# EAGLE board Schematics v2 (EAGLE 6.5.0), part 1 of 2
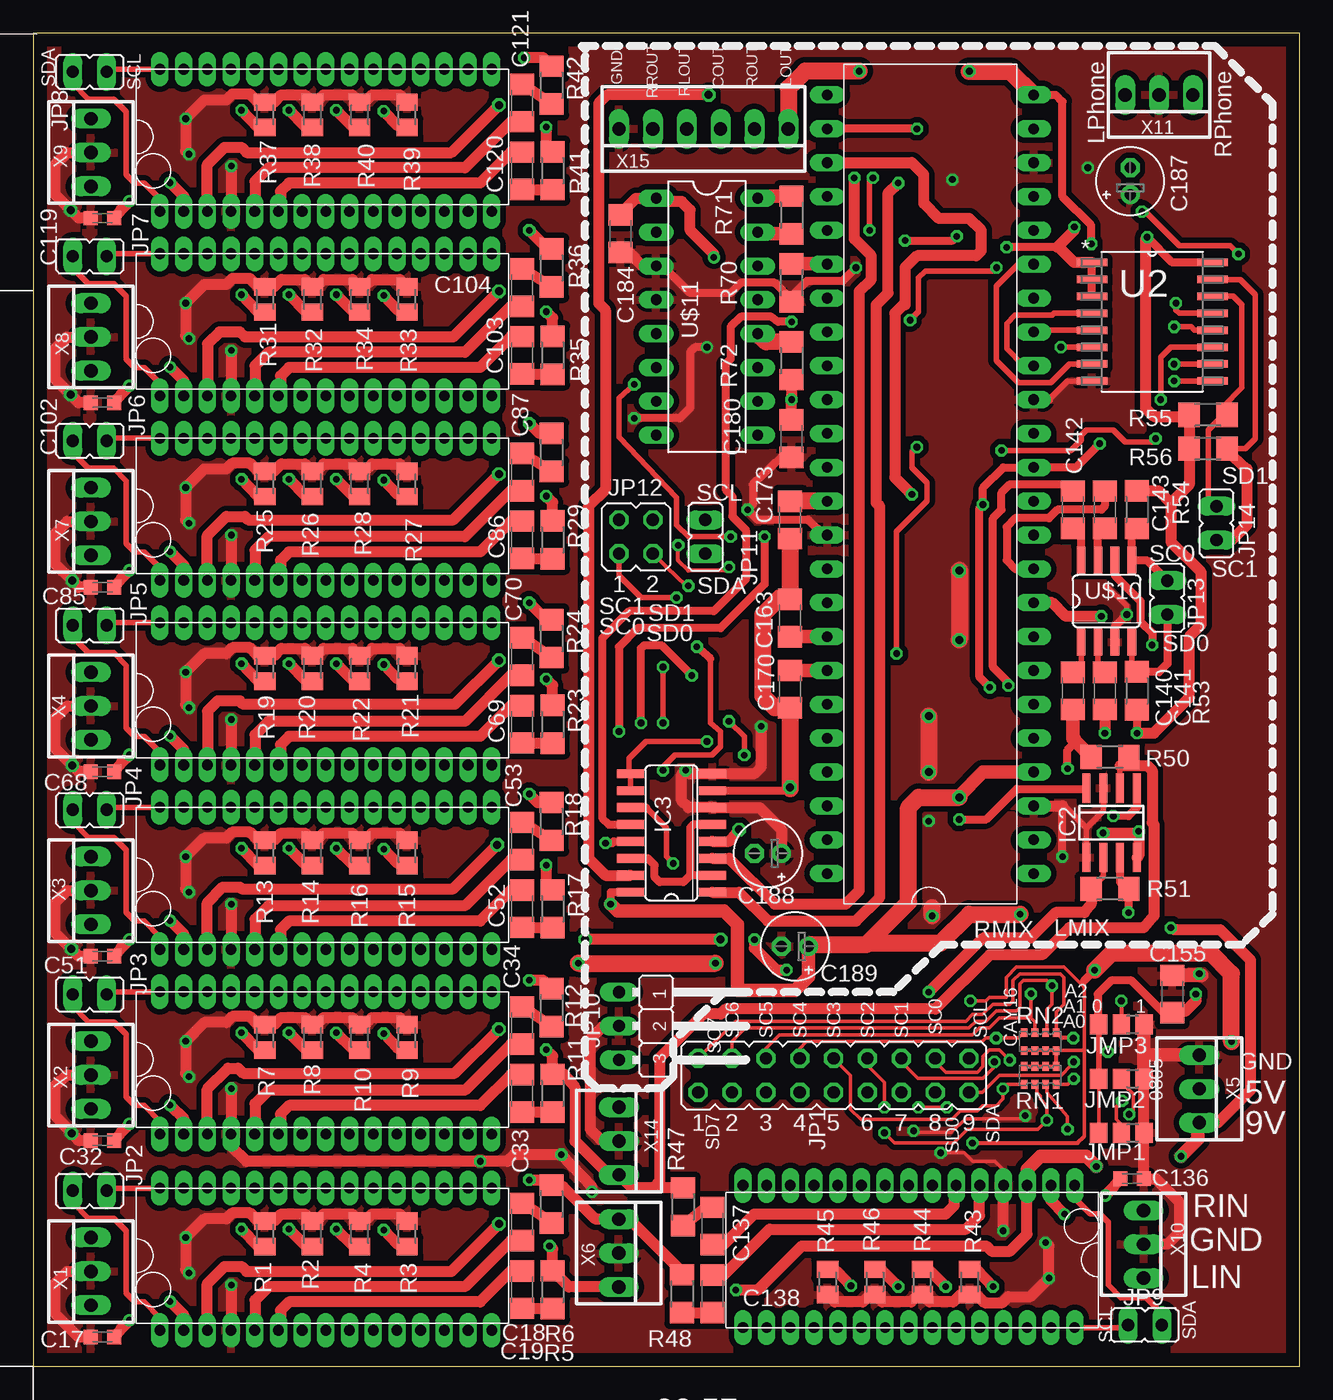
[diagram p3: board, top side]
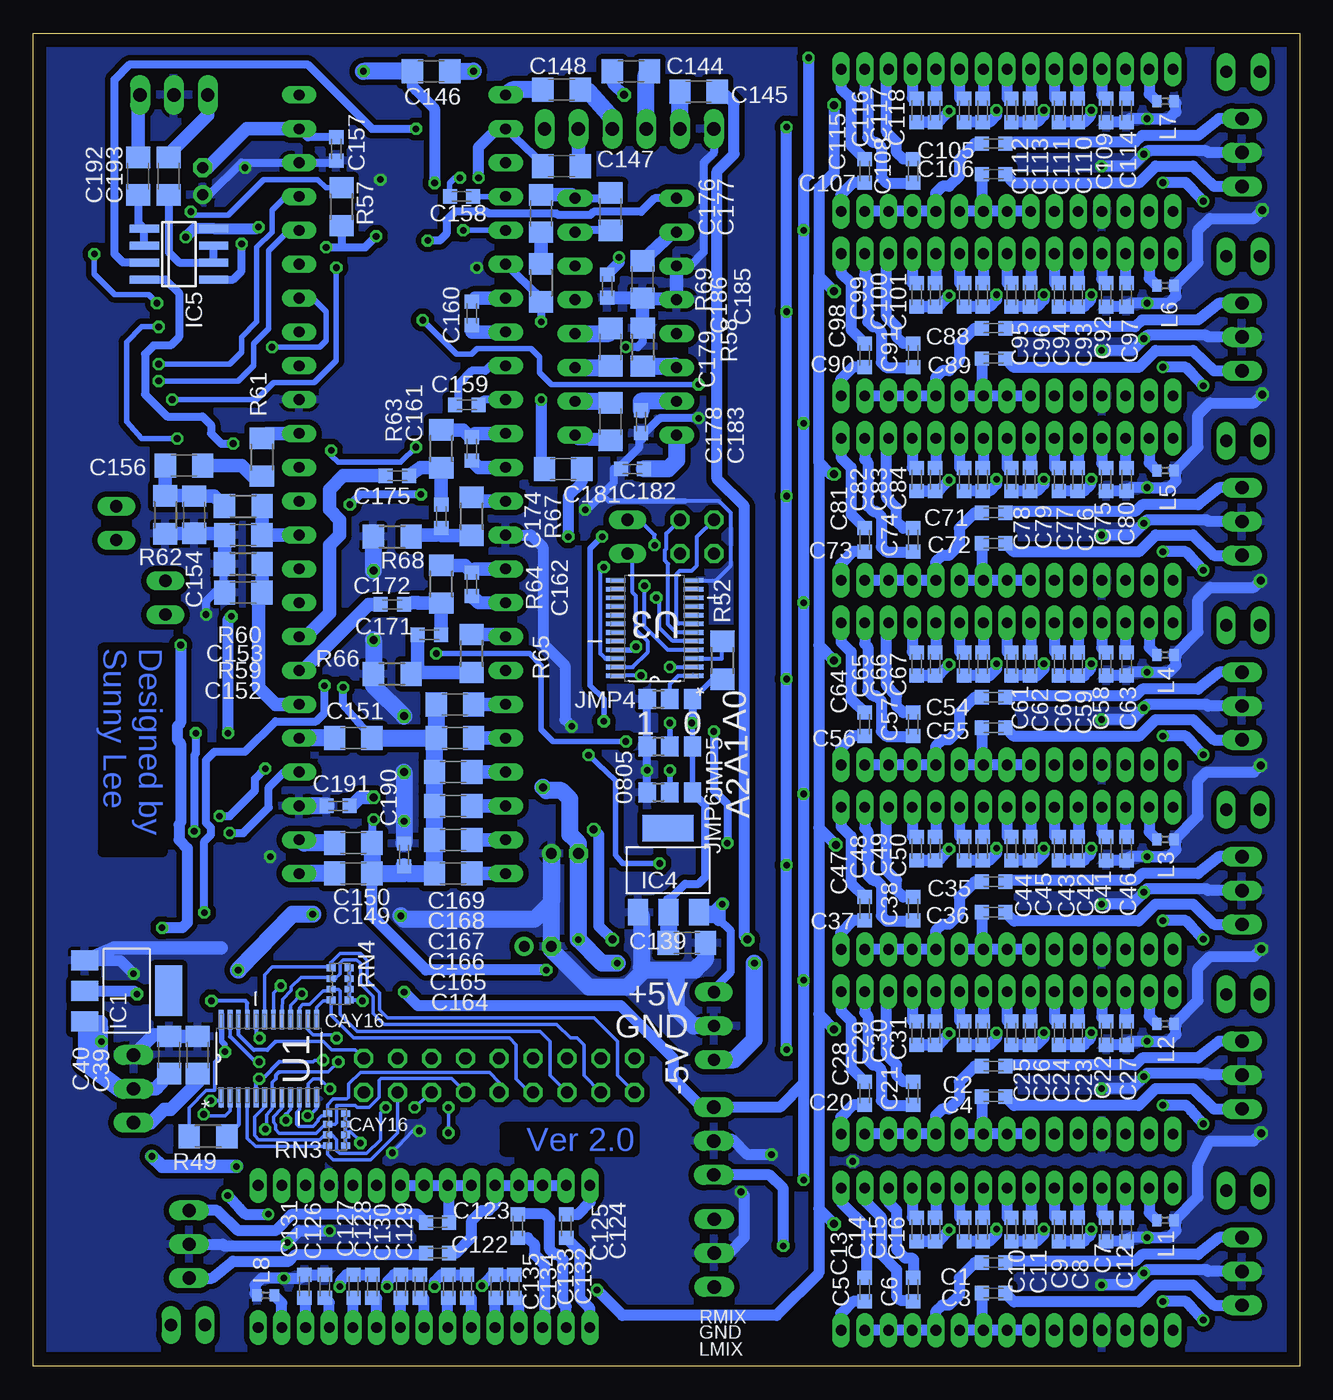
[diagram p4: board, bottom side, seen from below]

Size 95 x 100 mm. Coordinates in mm from the lower left corner, seen from the top.
Outline: 0,0 95,0 95,100 0,100 0,0
Copper layers (1*16): Top 0.035mm / dielectric 1.5mm / Bottom 0.035mm
Design rules "default *": minimum track width 10mil, minimum drill 0.4mm, track to track 0.1mm, track to pad 0.1mm, pad to pad 0.1mm, via to via 0.1mm, smd to smd 0.1mm, copper to edge 40mil, drill to drill 8mil, minimum pad ring 10mil, minimum via ring 8mil, stop-mask expansion 4mil, vias tented up to drill 0mil, thermal gap 10mil

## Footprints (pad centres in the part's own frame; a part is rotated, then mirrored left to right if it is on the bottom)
C0603K = smd 1.05 x 1.08: 1 -0.875,0; 2 0.875,0
C1206 = smd 1.6 x 1.8: 1 -1.4,0; 2 1.4,0
E2-5 = drill 0.813 pad 1.422: + -1.016,0 | drill 0.813 pad 1.422 octagon: - 1.016,0
SOT223 = smd 1.499 x 2.007: 1 -2.261,-3.15; 2 0.025,-3.15; 3 2.311,-3.15 | smd 3.81 x 2.007: 4 0,3.15
SO08 = smd 0.6 x 2.2: 1 -1.905,-2.6; 2 -0.635,-2.6; 3 0.635,-2.6; 4 1.905,-2.6; 5 1.905,2.6; 6 0.635,2.6; 7 -0.635,2.6; 8 -1.905,2.6
SO16 = smd 0.66 x 2.032: 1 -4.445,-3.073; 2 -3.175,-3.073; 3 -1.905,-3.073; 4 -0.635,-3.073; 5 0.635,-3.073; 6 1.905,-3.073; 7 3.175,-3.073; 8 4.445,-3.073; 9 4.445,3.073; 10 3.175,3.073; 11 1.905,3.073; 12 0.635,3.073; 13 -0.635,3.073; 14 -1.905,3.073; 15 -3.175,3.073; 16 -4.445,3.073
B0R-JMP = smd 1.5 x 1.3: 1 0,1.7; 2 0,0; 3 0,-1.7
JP9Q = drill 0.914 octagon: 1 -10.16,-1.27; 2 -10.16,1.27; 3 -7.62,-1.27; 4 -7.62,1.27; 5 -5.08,-1.27; 6 -5.08,1.27; 7 -2.54,-1.27; 8 -2.54,1.27; 9 0,-1.27; 10 0,1.27; 11 2.54,-1.27; 12 2.54,1.27; 13 5.08,-1.27; 14 5.08,1.27; 15 7.62,-1.27; 16 7.62,1.27; 17 10.16,-1.27; 18 10.16,1.27
JP1 = drill 0.914 long: 1 0,-1.27; 2 0,1.27
JP2W = drill 0.914 long: 1 -2.54,-1.27; 2 0,-1.27; 3 2.54,-1.27
JP2Q = drill 0.914 octagon: 1 -1.27,-1.27; 2 1.27,-1.27; 3 -1.27,1.27; 4 1.27,1.27
0402 = smd 0.7 x 0.9: 1 -0.65,0; 2 0.65,0
M0805 = smd 1.3 x 1.6: 1 -0.95,0; 2 0.95,0
R1206 = smd 1.6 x 1.803: 1 -1.422,0; 2 1.422,0
CAY16 = smd 0.5 x 0.65: 1 -1.2,-0.675; 2 -0.4,-0.675; 3 0.4,-0.675; 4 1.2,-0.675; 5 1.2,0.675; 6 0.4,0.675; 7 -0.4,0.675; 8 -1.2,0.675
SOP65P640X120-24N = smd 1.473 x 0.356: 1 -2.921,3.581; 2 -2.921,2.921; 3 -2.921,2.286; 4 -2.921,1.626; 5 -2.921,0.965; 6 -2.921,0.33; 7 -2.921,-0.33; 8 -2.921,-0.965; 9 -2.921,-1.626; 10 -2.921,-2.286; 11 -2.921,-2.921; 12 -2.921,-3.581; 13 2.921,-3.581; 14 2.921,-2.921; 15 2.921,-2.286; 16 2.921,-1.626; 17 2.921,-0.965; 18 2.921,-0.33; 19 2.921,0.33; 20 2.921,0.965; 21 2.921,1.626; 22 2.921,2.286; 23 2.921,2.921; 24 2.921,3.581
SOIC127P1032X265-16N = smd 2.286 x 0.559: 1 -4.521,4.445; 2 -4.521,3.175; 3 -4.521,1.905; 4 -4.521,0.635; 5 -4.521,-0.635; 6 -4.521,-1.905; 7 -4.521,-3.175; 8 -4.521,-4.445; 9 4.521,-4.445; 10 4.521,-3.175; 11 4.521,-1.905; 12 4.521,-0.635; 13 4.521,0.635; 14 4.521,1.905; 15 4.521,3.175; 16 4.521,4.445
SDIP30 = drill 0.8 long: P$1 1.778,-10.668; P$2 3.556,-10.668; P$3 5.334,-10.668; P$4 7.112,-10.668; P$5 8.89,-10.668; P$6 10.668,-10.668; P$7 12.446,-10.668; P$8 14.224,-10.668; P$9 16.002,-10.668; P$10 17.78,-10.668; P$11 19.558,-10.668; P$12 21.336,-10.668; P$13 23.114,-10.668; P$14 24.892,-10.668; P$15 26.67,-10.668; P$16 26.67,0; P$17 24.892,0; P$18 23.114,0; P$19 21.336,0; P$20 19.558,0; P$21 17.78,0; P$22 16.002,0; P$23 14.224,0; P$24 12.446,0; P$25 10.668,0; P$26 8.89,0; P$27 7.112,0; P$28 5.334,0; P$29 3.556,0; P$30 1.778,0
DIP48 = drill 0.8 long: P$1 -29.21,-8.89; P$2 -26.67,-8.89; P$3 -24.13,-8.89; P$4 -21.59,-8.89; P$5 -19.05,-8.89; P$6 -16.51,-8.89; P$7 -13.97,-8.89; P$8 -11.43,-8.89; P$9 -8.89,-8.89; P$10 -6.35,-8.89; P$11 -3.81,-8.89; P$12 -1.27,-8.89; P$13 1.27,-8.89; P$14 3.81,-8.89; P$15 6.35,-8.89; P$16 8.89,-8.89; P$17 11.43,-8.89; P$18 13.97,-8.89; P$19 16.51,-8.89; P$20 19.05,-8.89; P$21 21.59,-8.89; P$22 24.13,-8.89; P$23 26.67,-8.89; P$24 29.21,-8.89; P$25 29.21,6.604; P$26 26.67,6.604; P$27 24.13,6.604; P$28 21.59,6.604; P$29 19.05,6.604; P$30 16.51,6.604; P$31 13.97,6.604; P$32 11.43,6.604; P$33 8.89,6.604; P$34 6.35,6.604; P$35 3.81,6.604; P$36 1.27,6.604; P$37 -1.27,6.604; P$38 -3.81,6.604; P$39 -6.35,6.604; P$40 -8.89,6.604; P$41 -11.43,6.604; P$42 -13.97,6.604; P$43 -16.51,6.604; P$44 -19.05,6.604; P$45 -21.59,6.604; P$46 -24.13,6.604; P$47 -26.67,6.604; P$48 -29.21,6.604
SO08' = smd 0.66 x 2.032: 1 -1.905,-3.073; 2 -0.635,-3.073; 3 0.635,-3.073; 4 1.905,-3.073; 5 1.905,3.073; 6 0.635,3.073; 7 -0.635,3.073; 8 -1.905,3.073
DIL16 = drill 0.813 long: 1 -8.89,-3.81; 2 -6.35,-3.81; 3 -3.81,-3.81; 4 -1.27,-3.81; 5 1.27,-3.81; 6 3.81,-3.81; 7 6.35,-3.81; 8 8.89,-3.81; 9 8.89,3.81; 10 6.35,3.81; 11 3.81,3.81; 12 1.27,3.81; 13 -1.27,3.81; 14 -3.81,3.81; 15 -6.35,3.81; 16 -8.89,3.81
22-23-2031 = drill 1 long: 1 -2.54,0; 2 0,0; 3 2.54,0
22-23-2061 = drill 1 long: 1 -6.35,0; 2 -3.81,0; 3 -1.27,0; 4 1.27,0; 5 3.81,0; 6 6.35,0

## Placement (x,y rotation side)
C1  0.47u  [C0603K]  22.96,7.77 180 bottom
C2  0.47u  [C0603K]  22.96,22.5 180 bottom
C3  0.47u  [C0603K]  22.96,5.49 180 bottom
C4  0.47u  [C0603K]  22.96,20.22 180 bottom
C5  2.2u  [C0603K]  32.61,5.74 90 bottom
C6  2.2u  [C0603K]  28.98,5.74 90 bottom
C7  5.6n  [C0603K]  14.5,10.26 270 bottom
C8  18n  [C0603K]  16.66,10.26 270 bottom
C9  22n  [C0603K]  18.06,10.26 270 bottom
C10  100n  [C0603K]  21.62,10.26 270 bottom
C11  100n  [C0603K]  20.22,10.26 270 bottom
C12  5.6n  [C0603K]  12.98,10.26 270 bottom
C13  18n  [C0603K]  28.73,10.26 270 bottom
C14  22n  [C0603K]  27.33,10.26 270 bottom
C15  100n  [C0603K]  25.17,10.26 270 bottom
C16  100n  [C0603K]  23.77,10.26 270 bottom
C17  10u  [C0603K]  5.18,2.18 180 top
C18  10u  [C1206]  36.68,5.74 270 top
C19  10u  [C1206]  36.68,10.82 90 top
C20  2.2u  [C0603K]  32.61,20.47 90 bottom
C21  2.2u  [C0603K]  28.98,20.47 90 bottom
C22  5.6n  [C0603K]  14.5,24.99 270 bottom
C23  18n  [C0603K]  16.66,24.99 270 bottom
C24  22n  [C0603K]  18.06,24.99 270 bottom
C25  100n  [C0603K]  21.62,24.99 270 bottom
C26  100n  [C0603K]  20.22,24.99 270 bottom
C27  5.6n  [C0603K]  12.98,24.99 270 bottom
C28  18n  [C0603K]  28.73,24.99 270 bottom
C29  22n  [C0603K]  27.33,24.99 270 bottom
C30  100n  [C0603K]  25.17,24.99 270 bottom
C31  100n  [C0603K]  23.77,24.99 270 bottom
C32  10u  [C0603K]  5.18,16.92 180 top
C33  10u  [C1206]  36.68,20.47 270 top
C34  10u  [C1206]  36.68,25.55 90 top
C35  0.47u  [C0603K]  22.96,36.35 180 bottom
C36  0.47u  [C0603K]  22.96,34.06 180 bottom
C37  2.2u  [C0603K]  32.61,34.32 90 bottom
C38  2.2u  [C0603K]  28.98,34.32 90 bottom
C39  10u  [C1206]  82.65,23.34 90 bottom
C40  10u  [C1206]  84.81,23.34 90 bottom
C41  5.6n  [C0603K]  14.5,38.84 270 bottom
C42  18n  [C0603K]  16.66,38.84 270 bottom
C43  22n  [C0603K]  18.06,38.84 270 bottom
C44  100n  [C0603K]  21.62,38.84 270 bottom
C45  100n  [C0603K]  20.22,38.84 270 bottom
C46  5.6n  [C0603K]  12.98,38.84 270 bottom
C47  18n  [C0603K]  28.73,38.84 270 bottom
C48  22n  [C0603K]  27.33,38.84 270 bottom
C49  100n  [C0603K]  25.17,38.84 270 bottom
C50  100n  [C0603K]  23.77,38.84 270 bottom
C51  10u  [C0603K]  5.18,30.76 180 top
C52  10u  [C1206]  36.68,34.32 270 top
C53  10u  [C1206]  36.68,39.4 90 top
C54  0.47u  [C0603K]  22.96,50.19 180 bottom
C55  0.47u  [C0603K]  22.96,47.9 180 bottom
C56  2.2u  [C0603K]  32.61,48.16 90 bottom
C57  2.2u  [C0603K]  28.98,48.16 90 bottom
C58  5.6n  [C0603K]  14.5,52.68 270 bottom
C59  18n  [C0603K]  16.66,52.68 270 bottom
C60  22n  [C0603K]  18.06,52.68 270 bottom
C61  100n  [C0603K]  21.62,52.68 270 bottom
C62  100n  [C0603K]  20.22,52.68 270 bottom
C63  5.6n  [C0603K]  12.98,52.68 270 bottom
C64  18n  [C0603K]  28.73,52.68 270 bottom
C65  22n  [C0603K]  27.33,52.68 270 bottom
C66  100n  [C0603K]  25.17,52.68 270 bottom
C67  100n  [C0603K]  23.77,52.68 270 bottom
C68  10u  [C0603K]  5.18,44.6 180 top
C69  10u  [C1206]  36.68,48.16 270 top
C70  10u  [C1206]  36.68,53.24 90 top
C71  0.47u  [C0603K]  22.96,64.03 180 bottom
C72  0.47u  [C0603K]  22.96,61.75 180 bottom
C73  2.2u  [C0603K]  32.61,62 90 bottom
C74  2.2u  [C0603K]  28.98,62 90 bottom
C75  5.6n  [C0603K]  14.5,66.52 270 bottom
C76  18n  [C0603K]  16.66,66.52 270 bottom
C77  22n  [C0603K]  18.06,66.52 270 bottom
C78  100n  [C0603K]  21.62,66.52 270 bottom
C79  100n  [C0603K]  20.22,66.52 270 bottom
C80  5.6n  [C0603K]  12.98,66.52 270 bottom
C81  18n  [C0603K]  28.73,66.52 270 bottom
C82  22n  [C0603K]  27.33,66.52 270 bottom
C83  100n  [C0603K]  25.17,66.52 270 bottom
C84  100n  [C0603K]  23.77,66.52 270 bottom
C85  10u  [C0603K]  5.18,58.45 180 top
C86  10u  [C1206]  36.68,62 270 top
C87  10u  [C1206]  36.68,67.08 90 top
C88  0.47u  [C0603K]  22.96,77.88 180 bottom
C89  0.47u  [C0603K]  22.96,75.59 180 bottom
C90  2.2u  [C0603K]  32.61,75.84 90 bottom
C91  2.2u  [C0603K]  28.98,75.84 90 bottom
C92  5.6n  [C0603K]  14.5,80.37 270 bottom
C93  18n  [C0603K]  16.66,80.37 270 bottom
C94  22n  [C0603K]  18.06,80.37 270 bottom
C95  100n  [C0603K]  21.62,80.37 270 bottom
C96  100n  [C0603K]  20.22,80.37 270 bottom
C97  5.6n  [C0603K]  12.98,80.37 270 bottom
C98  18n  [C0603K]  28.73,80.37 270 bottom
C99  22n  [C0603K]  27.33,80.37 270 bottom
C100  100n  [C0603K]  25.17,80.37 270 bottom
C101  100n  [C0603K]  23.77,80.37 270 bottom
C102  10u  [C0603K]  5.18,72.29 180 top
C103  10u  [C1206]  36.68,75.84 270 top
C104  10u  [C1206]  36.68,80.92 90 top
C105  0.47u  [C0603K]  22.96,91.72 180 bottom
C106  0.47u  [C0603K]  22.96,89.43 180 bottom
C107  2.2u  [C0603K]  32.61,89.69 90 bottom
C108  2.2u  [C0603K]  28.98,89.69 90 bottom
C109  5.6n  [C0603K]  14.5,94.21 270 bottom
C110  18n  [C0603K]  16.66,94.21 270 bottom
C111  22n  [C0603K]  18.06,94.21 270 bottom
C112  100n  [C0603K]  21.62,94.21 270 bottom
C113  100n  [C0603K]  20.22,94.21 270 bottom
C114  5.6n  [C0603K]  12.98,94.21 270 bottom
C115  18n  [C0603K]  28.73,94.21 270 bottom
C116  22n  [C0603K]  27.33,94.21 270 bottom
C117  100n  [C0603K]  25.17,94.21 270 bottom
C118  100n  [C0603K]  23.77,94.21 270 bottom
C119  10u  [C0603K]  5.18,86.13 180 top
C120  10u  [C1206]  36.68,89.69 270 top
C121  10u  [C1206]  36.68,94.77 90 top
C122  0.47u  [C0603K]  64.67,8.48 0 bottom
C123  0.47u  [C0603K]  64.67,10.77 0 bottom
C124  2.2u  [C0603K]  55.02,10.52 270 bottom
C125  2.2u  [C0603K]  58.65,10.52 270 bottom
C126  5.6n  [C0603K]  73.13,5.99 90 bottom
C127  18n  [C0603K]  70.97,5.99 90 bottom
C128  22n  [C0603K]  69.57,5.99 90 bottom
C129  100n  [C0603K]  66.01,5.99 90 bottom
C130  100n  [C0603K]  67.41,5.99 90 bottom
C131  5.6n  [C0603K]  74.65,5.99 90 bottom
C132  18n  [C0603K]  58.9,5.99 90 bottom
C133  22n  [C0603K]  60.3,5.99 90 bottom
C134  100n  [C0603K]  62.46,5.99 90 bottom
C135  100n  [C0603K]  63.86,5.99 90 bottom
C136  10u  [C0603K]  82.45,14.07 0 top
C137  10u  [C1206]  50.95,10.52 90 top
C138  10u  [C1206]  50.95,5.44 270 top
C139  10u  [C1206]  45.97,31.75 0 bottom
C140  10u  [C1206]  77.98,50.67 270 top
C141  10u  [C1206]  80.39,50.67 270 top
C142  10u  [C1206]  77.98,64.26 90 top
C143  10u  [C1206]  80.39,64.26 90 top
C144  10u  [C1206]  50.16,97.16 0 bottom
C145  10u  [C1206]  45.09,95.63 180 bottom
C146  10u  [C1206]  65.15,97.16 0 bottom
C147  10u  [C1206]  55.37,90.04 0 bottom
C148  10u  [C1206]  55.37,95.76 0 bottom
C149  4.7u  [C1206]  70.99,36.96 0 bottom
C150  0.22u  [C1206]  70.99,39.24 0 bottom
C151  0.22u  [C1206]  70.99,47.12 0 bottom
C152  10u  [C1206]  79.25,58.04 180 bottom
C153  10n  [C1206]  79.25,62.36 180 bottom
C154  10n  [C1206]  82.93,63.88 270 bottom
C155  10u  [C1206]  85.45,27.91 90 top
C156  10n  [C1206]  83.69,67.56 180 bottom
C157  100n  [C0603K]  72.26,91.31 270 bottom
C158  100n  [C0603K]  62.87,87.76 180 bottom
C159  22n  [C0603K]  62.48,72.14 0 bottom
C160  22n  [C0603K]  62.1,78.99 270 bottom
C161  22n  [C0603K]  62.1,68.83 270 bottom
C162  22n  [C0603K]  62.1,58.67 270 bottom
C163  680p  [C1206]  56.77,56.13 270 top
C164  4.7u  [C1206]  63.5,36.96 0 bottom
C165  0.22u  [C1206]  63.5,39.5 0 bottom
C166  0.22u  [C1206]  63.5,42.04 0 bottom
C167  0.33u  [C1206]  63.5,44.58 0 bottom
C168  0.33u  [C1206]  63.37,47.12 0 bottom
C169  0.33u  [C1206]  63.37,49.66 0 bottom
C170  0.33u  [C1206]  56.77,50.8 90 top
C171  100n  [C0603K]  65.28,54.86 180 bottom
C172  100n  [C0603K]  68.07,57.15 0 bottom
C173  680p  [C1206]  56.77,63.5 90 top
C174  100n  [C0603K]  64.39,63.75 270 bottom
C175  100n  [C0603K]  67.69,66.8 0 bottom
C176  10u  [C1206]  56.9,86.49 270 bottom
C177  1n  [C1206]  51.69,86.61 90 bottom
C178  10n  [C1206]  51.69,70.87 270 bottom
C179  10n  [C1206]  51.69,76.45 270 bottom
C180  10n  [C1206]  56.9,69.6 270 top
C181  10u  [C1206]  55.24,67.31 0 bottom
C182  100n  [C0603K]  50.04,67.31 180 bottom
C183  100n  [C0603K]  49.4,70.87 270 bottom
C184  10u  [C1206]  44.07,84.96 270 top
C185  10u  [C1206]  49.28,81.53 270 bottom
C186  100n  [C0603K]  51.94,81.03 270 bottom
C187  100u  [E2-5]  82.3,88.9 90 top
C188  100u  [E2-5]  55.12,38.48 180 top
C189  100u  [E2-5]  57.15,31.5 180 top
C190  100n  [C0603K]  67.18,38.35 270 bottom
C191  100n  [C0603K]  72.14,42.04 180 bottom
C192  10u  [C1206]  87.12,89.28 90 bottom
C193  10u  [C1206]  84.84,89.28 90 bottom
IC1  REG1117  [SOT223]  87.99,28.17 270 bottom
IC2  LM358D  [SO08]  80.9,40.77 180 top
IC3  4053D  [SO16]  47.88,40.01 90 top
IC4  REG1117  [SOT223]  47.37,37.21 0 bottom
IC5  LM358D  [SO08]  84.07,83.44 270 bottom
JMP1  0R-JUMPB  [B0R-JMP]  81.64,17.5 90 top
JMP2  0R-JUMPB  [B0R-JMP]  81.64,21.56 90 top
JMP3  0R-JUMPB  [B0R-JMP]  81.64,25.63 90 top
JMP4  0R-JUMPB  [B0R-JMP]  47.24,50.04 270 bottom
JMP5  0R-JUMPB  [B0R-JMP]  47.24,46.48 270 bottom
JMP6  0R-JUMPB  [B0R-JMP]  47.24,43.05 270 bottom
JP1  [JP9Q]  60.05,21.82 0 top
JP2  [JP1]  4.23,13.17 90 top
JP3  [JP1]  4.23,27.9 90 top
JP4  [JP1]  4.23,41.74 90 top
JP5  [JP1]  4.23,55.59 90 top
JP6  [JP1]  4.23,69.43 90 top
JP7  [JP1]  4.23,83.27 90 top
JP8  [JP1]  4.23,97.12 90 top
JP9  [JP1]  83.4,3.09 270 top
JP10  [JP2W]  45.21,25.53 270 top
JP11  [JP1]  50.42,62.23 0 top
JP12  [JP2Q]  45.21,62.23 0 top
JP13  [JP1]  85.09,57.66 180 top
JP14  [JP1]  88.77,63.25 180 top
L1  BLM15HB121SN1  [0402]  10.06,10.95 0 bottom
L2  BLM15HB121SN1  [0402]  10.06,25.68 0 bottom
L3  BLM15HB121SN1  [0402]  10.06,39.52 0 bottom
L4  BLM15HB121SN1  [0402]  10.06,53.37 0 bottom
L5  BLM15HB121SN1  [0402]  10.06,67.21 0 bottom
L6  BLM15HB121SN1  [0402]  10.06,81.05 0 bottom
L7  BLM15HB121SN1  [0402]  10.06,94.89 0 bottom
L8  BLM15HB121SN1  [0402]  77.57,5.31 180 bottom
R1  2.7k  [M0805]  17.37,9.93 90 top
R2  5.6k  [M0805]  20.93,9.93 90 top
R3  2.7k  [M0805]  28.04,9.93 270 top
R4  5.6k  [M0805]  24.49,9.93 270 top
R5  10k  [R1206]  38.96,5.74 90 top
R6  10k  [R1206]  38.89,12.17 90 top
R7  2.7k  [M0805]  17.37,24.66 90 top
R8  5.6k  [M0805]  20.93,24.66 90 top
R9  2.7k  [M0805]  28.04,24.66 270 top
R10  5.6k  [M0805]  24.49,24.66 270 top
R11  10k  [R1206]  38.96,20.47 90 top
R12  10k  [R1206]  38.89,26.9 90 top
R13  2.7k  [M0805]  17.37,38.51 90 top
R14  5.6k  [M0805]  20.93,38.51 90 top
R15  2.7k  [M0805]  28.04,38.51 270 top
R16  5.6k  [M0805]  24.49,38.51 270 top
R17  10k  [R1206]  38.96,34.32 90 top
R18  10k  [R1206]  38.89,40.87 90 top
R19  2.7k  [M0805]  17.37,52.35 90 top
R20  5.6k  [M0805]  20.93,52.35 90 top
R21  2.7k  [M0805]  28.04,52.35 270 top
R22  5.6k  [M0805]  24.49,52.35 270 top
R23  10k  [R1206]  38.96,48.16 90 top
R24  10k  [R1206]  38.89,54.58 90 top
R25  2.7k  [M0805]  17.37,66.19 90 top
R26  5.6k  [M0805]  20.93,66.19 90 top
R27  2.7k  [M0805]  28.04,66.19 270 top
R28  5.6k  [M0805]  24.49,66.19 270 top
R29  10k  [R1206]  38.96,62 90 top
R30  10k  [R1206]  38.89,68.55 90 top
R31  2.7k  [M0805]  17.37,80.04 90 top
R32  5.6k  [M0805]  20.93,80.04 90 top
R33  2.7k  [M0805]  28.04,80.04 270 top
R34  5.6k  [M0805]  24.49,80.04 270 top
R35  10k  [R1206]  38.96,75.84 90 top
R36  10k  [R1206]  38.89,82.4 90 top
R37  2.7k  [M0805]  17.37,93.88 90 top
R38  5.6k  [M0805]  20.93,93.88 90 top
R39  2.7k  [M0805]  28.04,93.88 270 top
R40  5.6k  [M0805]  24.49,93.88 270 top
R41  10k  [R1206]  38.96,89.69 90 top
R42  10k  [R1206]  38.89,96.11 90 top
R43  2.7k  [M0805]  70.26,6.32 270 top
R44  5.6k  [M0805]  66.7,6.32 270 top
R45  2.7k  [M0805]  59.59,6.32 90 top
R46  5.6k  [M0805]  63.14,6.32 90 top
R47  10k  [R1206]  48.74,11.96 90 top
R48  10k  [R1206]  48.67,5.44 90 top
R49  10k  [R1206]  81.89,17.25 0 bottom
R50  10k  [R1206]  80.77,45.72 180 top
R51  10k  [R1206]  80.77,35.81 0 top
R52  10k  [R1206]  43.31,52.96 90 bottom
R53  10k  [R1206]  82.8,50.67 90 top
R54  10k  [R1206]  82.8,64.26 90 top
R55  10k  [R1206]  88.14,71.37 0 top
R56  10k  [R1206]  88.14,68.83 0 top
R57  10k  [R1206]  71.88,87 90 bottom
R58  2.2k  [R1206]  49.28,76.45 90 bottom
R59  10M  [R1206]  79.25,60.2 180 bottom
R60  22k  [R1206]  79.25,64.52 180 bottom
R61  22k  [R1206]  77.85,68.2 90 bottom
R62  22k  [R1206]  85.09,63.88 90 bottom
R63  7.5k  [R1206]  64.39,68.83 270 bottom
R64  7.5k  [R1206]  64.39,58.67 270 bottom
R65  47k  [R1206]  62.1,53.47 270 bottom
R66  15k  [R1206]  68.07,51.94 180 bottom
R67  47k  [R1206]  62.1,63.75 270 bottom
R68  15k  [R1206]  68.07,62.23 180 bottom
R69  10k  [R1206]  56.9,81.28 90 bottom
R70  10k  [R1206]  56.9,81.28 270 top
R71  10k  [R1206]  56.9,86.36 90 top
R72  1k  [R1206]  56.9,75.44 90 top
RN1  [CAY16]  75.54,21.82 180 top
RN2  [CAY16]  75.54,24.36 0 top
RN3  [CAY16]  72.24,17.75 270 bottom
RN4  [CAY16]  71.98,28.68 270 bottom
U1  PCA9548APWR  [SOP65P640X120-24N]  77.32,23.09 90 bottom
U2  PCF8574AT/3,512  [SOIC127P1032X265-16N]  83.95,78.36 0 top
U3  PCA9548APWR  [SOP65P640X120-24N]  48.39,55.37 180 bottom
U$1  TDA7439  [SDIP30]  7.72,13.36 0 top
U$2  TDA7439  [SDIP30]  7.72,28.09 0 top
U$3  TDA7439  [SDIP30]  7.72,41.94 0 top
U$4  TDA7439  [SDIP30]  7.72,55.78 0 top
U$5  TDA7439  [SDIP30]  7.72,69.62 0 top
U$6  TDA7439  [SDIP30]  7.72,83.46 0 top
U$7  TDA7439  [SDIP30]  7.72,97.31 0 top
U$8  TDA7439  [SDIP30]  79.91,2.9 180 top
U$9  SSM2126  [DIP48]  66.17,66.17 90 top
U$10  PT2257  [SO08']  80.52,57.4 0 top
U$11  PT2399  [DIL16]  50.55,78.74 270 top
X1  22-23-2031  [22-23-2031]  4.32,7.11 90 top
X2  22-23-2031  [22-23-2031]  4.32,21.84 90 top
X3  22-23-2031  [22-23-2031]  4.32,35.69 90 top
X4  22-23-2031  [22-23-2031]  4.32,49.53 90 top
X5  22-23-2031  [22-23-2031]  87.48,20.8 270 top
X6  22-23-2031  [22-23-2031]  43.92,8.48 270 top
X7  22-23-2031  [22-23-2031]  4.32,63.37 90 top
X8  22-23-2031  [22-23-2031]  4.32,77.22 90 top
X9  22-23-2031  [22-23-2031]  4.32,91.06 90 top
X10  22-23-2031  [22-23-2031]  83.31,9.14 270 top
X11  22-23-2031  [22-23-2031]  84.45,95.38 180 top
X14  22-23-2031  [22-23-2031]  43.94,16.89 270 top
X15  [22-23-2061]  50.29,92.84 180 top

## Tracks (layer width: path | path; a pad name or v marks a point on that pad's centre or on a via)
3.3V  (via drill 0.5)
  Top 0.254: JMP2.1 JMP1.1
  Top 0.305: C155.1 84.81,26.52 | 79.86,25.71 JMP3.1
  Top 0.406: JMP2.1 79.94,23.34 | 79.94,23.34 JMP3.1 | v80.62,23.6 80.19,23.6 79.94,23.34
  Top 0.61: 84.81,26.52 82.4,28.93 80.87,28.93 79.86,27.91 79.86,25.71
  Top 0.813: v87.22,27.91 87.22,27.41 86.46,26.64 85.58,26.64 C155.1
  Bottom 0.254: R49.1 83.31,19.38 82.02,20.68 81.38,20.68 81.38,22.84 v80.62,23.6
  Bottom 0.406: U1.24 80.9,26.36 80.87,26.39 80.87,24.36 80.62,24.11 v80.62,23.6
  Bottom 0.813: IC1.2 87.45,28.14 v87.22,27.91
3.3V1  (via drill 0.5)
  Top 0.61: v45.59,48.26 45.59,53.85 45.85,54.1 47.12,54.1 v49.4,51.82
  Bottom 0.305: v49.4,51.82 51.28,51.82 U3.24
  Bottom 0.406: JMP6.1 JMP5.1 JMP4.1 44.05,51.54 R52.1
  Bottom 0.61: JMP6.1 44.58,42.09 44.58,36.7 45.09,36.2 46.1,36.2 47.35,34.95 | JMP4.1 45.54,48.31 v45.59,48.26
  Bottom 0.813: 47.35,34.95 IC4.2
  Bottom 1.27: IC4.2 47.35,31.78 C139.1
9V  (via drill 0.5, 0.6)
  Top 0.61: U$10.6 81.15,59.31 83.06,57.4 83.06,55.88 83.95,54.99 v83.95,54.1
  Top 0.813: U$7.P$3 13.06,90.14 14.35,91.44 15.62,91.44 16,91.06 31.37,91.06 v34.92,94.61 | v34.92,80.64 31.5,77.22 15.88,77.22 15.49,77.6 13.97,77.6 13.08,76.71 13.08,72.82 U$6.P$3 | U$5.P$3 13.06,62.33 14.48,63.75 15.88,63.75 16.13,63.5 31.5,63.5 v34.92,66.93 | v34.92,52.96 31.62,49.66 15.75,49.66 15.49,49.91 13.84,49.91 13.08,49.15 13.08,45.14 U$4.P$3 | U$3.P$3 13.06,34.77 14.22,35.94 15.49,35.94 15.62,35.81 31.5,35.81 v34.8,39.12 | U$2.P$3 13.06,20.8 14.61,22.35 15.37,22.35 15.75,21.97 31.62,21.97 v34.92,25.27 | U$1.P$3 13.06,6.2 14.35,7.49 15.62,7.49 16,7.11 31.37,7.11 v34.92,10.67 | v85.34,32.89 85.6,32.77 89.03,32.77 91.31,30.48 91.31,20.7 88.9,18.29 87.5,18.29 X5.3 | v52.7,5.71 54.36,5.71 57.66,9.02 71.5,9.02 71.88,8.64 73.28,8.64 74.55,9.91 74.55,13.54 U$8.P$3
  Top 1.016: U$8.P$3 74.57,14.76 75.56,15.75 78.99,15.75 v79.76,14.99 | X5.3 87.38,18.16 87.38,17.02 v86.11,15.75
  Bottom 0.813: v34.92,94.61 34.92,89.53 36.07,88.39 36.07,81.79 | 36.07,81.79 v34.92,80.64 | v34.92,66.93 35.18,66.93 36.07,67.82 | 36.07,67.82 36.07,81.79 | 36.07,67.82 36.07,54.1 | 36.07,54.1 v34.92,52.96 | 36.07,54.1 36.07,40.39 | 36.07,40.39 v34.8,39.12 | 36.07,40.39 36.07,26.42 | 36.07,26.42 v34.92,25.27 | 36.07,26.42 36.07,11.81 | 36.07,11.81 v34.92,10.67 | v83.95,54.1 83.95,48.26 84.2,48.01 84.2,46.99 83.95,46.74 83.95,40.77 84.07,40.64 84.07,39.5 83.44,38.86 83.44,33.27 83.82,32.89 v85.34,32.89 | 36.07,11.81 36.07,6.99 39.24,3.81 50.8,3.81 v52.7,5.71
  Bottom 1.016: C39.1 82.65,21.31 84.68,19.28 85.19,19.28 86.21,18.26 X5.3 | v79.76,14.99 85.34,14.99 v86.11,15.75
BYPASS  (via drill 0.5)
  Top 0.406: IC3.10 IC3.9 | v50.55,46.86 45.97,46.86 44.7,45.59 44.7,44.55 | v64.77,53.47 64.77,62.61 67.06,64.9 67.06,66.29 65.91,67.44 65.91,68.58 v66.29,68.96 | v72.64,68.71 77.85,68.71 78.61,69.47 78.61,69.85 78.99,70.23 81.03,70.23 81.92,69.34 83.95,69.34 v84.2,69.6 | v85.6,77.98 86.87,77.98 87.12,77.72 U2.12
  Top 0.61: 44.7,44.55 IC3.9
  Bottom 0.406: v50.55,46.86 56.01,46.86 56.9,47.75 56.9,52.58 57.78,53.47 v64.77,53.47 | v66.29,68.96 67.44,67.82 72.14,67.82 72.64,68.33 v72.64,68.71 | v84.2,69.6 86.87,69.6 88.01,70.87 88.01,76.83 86.87,77.98 v85.6,77.98
CM1  (via drill 0.5)
  Top 0.406: v85.6,73.91 U2.9
  Bottom 0.406: U$9.P$20 75.82,85.22 77.34,83.69 77.34,77.85 78.49,76.71 78.49,75.06 79.63,73.91 v85.6,73.91
CM2  (via drill 0.5)
  Top 0.406: U2.10 v85.6,75.18
  Bottom 0.406: v85.6,75.18 80.26,75.18 79.38,76.07 79.38,77.22 78.23,78.36 78.23,83.95 77.09,85.09 77.09,86.74 76.07,87.76 U$9.P$21
COUT
  Bottom 1.27: C148.2 53.34,95.63 51.56,93.6 X15.3
DELAY  (via drill 0.5)
  Top 0.406: 45.97,41.91 47.5,40.39 47.5,38.23 v48.01,37.72 | v53.34,45.85 53.34,47.24 v52.2,48.39 | v52.32,62.23 49.15,62.23 48.26,63.12 48.26,65.15 43.94,69.72 43.94,72.64 v45.09,73.66 | U2.11 85.34,76.45 84.58,75.69 v84.58,72.52 | v72.26,82.42 72.01,82.17 66.93,82.17 66.42,81.66 66.42,79.12 v65.79,78.49
  Top 0.61: IC3.11 45.97,41.91
  Bottom 0.406: v45.09,73.66 56.13,73.66 57.02,74.55 57.02,75.69 57.66,76.33 61.72,76.33 62.1,75.95 63.25,75.95 v65.79,78.49 | v48.01,37.72 50.8,37.72 51.31,38.35 51.31,43.94 v53.34,45.85 | v52.2,48.39 52.2,50.04 53.21,51.05 53.21,61.34 v52.32,62.23 | v84.58,72.52 78.23,72.52 76.96,73.79 73.91,73.79 72.26,75.44 v72.26,82.42
DELFED  (via drill 0.5)
  Top 0.61: v54.86,62.23 54.86,58.67 51.56,55.37 45.34,55.37 43.94,53.98 v43.94,47.62 | v42.93,39.24 43.43,39.24 43.56,39.37 IC3.13
  Bottom 0.61: C181.2 53.84,66.42 | v43.94,47.62 43.94,43.18 42.93,42.16 v42.93,39.24
  Bottom 0.813: 53.84,66.42 53.84,66.3 54.86,65.28 v54.86,62.23
DM1
  Top 0.406: U2.4 76.58,78.99 76.45,78.87 73.66,78.87 73.03,78.23 73.03,76.33 74.3,75.06 U$9.P$16
DM2
  Top 0.406: U2.5 75.18,77.72 U$9.P$17
DM3  (via drill 0.5)
  Top 0.406: U2.6 v77.09,76.45
  Bottom 0.406: v77.09,76.45 73.53,76.45 73.03,76.96 73.03,79.12 74.04,80.14 U$9.P$18
DM4
  Top 0.406: U2.7 77.72,75.18 76.33,73.79 73.91,73.79 72.26,75.44 72.26,81.03 73.91,82.68 U$9.P$19
GND  (via drill 0.5, 0.6)
  Top 0.254: v74.42,18.8 74.17,18.54 69.98,18.54 68.83,17.53 66.17,17.53 v66.04,17.65 | v68.07,16 69.85,16 70.48,15.37 72.14,15.37 72.77,14.73 72.77,13.59 U$8.P$4
  Top 0.406: U$10.3 81.15,54.23 81.28,54.1 81.28,55.63 v82.04,56.39 82.04,57.02 80.52,58.55 | IC2.3 80.26,41.66 78.99,40.39 | 78.99,40.39 IC2.5 | 77.22,42.04 77.34,42.04 78.99,40.39 | U2.8 77.6,73.91 76.2,72.52
  Top 0.61: U$10.3 81.15,55.5 v82.04,56.39 | v77.22,38.23 77.22,42.04 | U$9.P$15 76.2,72.52 | v61.72,82.42 60.71,81.41 58.04,81.41 56.9,80.26 R70.2 56.9,80.01 55.63,81.28 53.09,81.28 52.32,80.52 49.28,80.52 47.24,82.55 | 48.64,44.4 v48.94,44.7 | IC3.8 50.42,44.45 | C180.2 56.13,68.2 53.98,66.17 53.98,64.64 v53.59,64.26 54.36,63.5 58.17,63.5 59.31,62.36 U$9.P$38 | v50.55,76.45 49.66,76.45 49.28,76.07 49.28,71.88 48.51,71.12 v45.09,71.12
  Top 0.813: R3.1 27.49,11.43 25.4,11.43 24.85,10.88 R4.1 23.94,11.43 21.78,11.43 21.23,10.88 R2.2 20.38,11.43 18.61,11.43 18.06,10.88 R1.2 16.87,10.88 16.26,11.49 14.92,11.49 14.48,11.05 12.83,11.05 v11.43,9.65 11.43,7.24 v11.68,6.99 | U$1.P$4 14.86,2.72 v14.86,6.1 | v87.48,29.44 85.57,29.44 C155.2 | JMP2.3 JMP1.3 83.32,17.49 C136.2 84.23,14.07 85.98,12.32 85.98,10.03 85.09,9.14 X10.2 | C17.2 3.4,2.18 1.65,3.94 1.65,6.22 2.54,7.11 X1.2 | R9.1 27.49,26.16 25.4,26.16 24.85,25.61 R10.1 23.94,26.16 21.78,26.16 21.23,25.61 R8.2 20.38,26.16 18.61,26.16 18.06,25.61 R7.2 16.87,25.61 16.26,26.23 14.92,26.23 14.48,25.78 12.83,25.78 v11.43,24.38 11.43,21.97 v11.68,21.72 | v14.86,20.83 14.86,17.45 U$2.P$4 14.86,17.4 14.86,16.51 16,15.37 v33.53,15.37 35.56,15.37 36.07,15.88 v39.62,15.88 41.91,13.46 v41.91,13.08 | C32.2 3.4,16.92 3.18,17.15 | 3.18,17.15 v2.88,17.48 | v2.88,17.48 1.65,18.8 1.65,21.08 2.54,21.84 X2.2 | R15.1 27.49,40.01 25.4,40.01 24.85,39.46 R16.1 23.94,40.01 21.78,40.01 21.23,39.46 R14.2 20.38,40.01 18.61,40.01 18.06,39.46 R13.2 16.87,39.46 16.26,40.07 14.92,40.07 14.48,39.62 12.83,39.62 v11.43,38.23 11.43,35.81 v11.68,35.56 | U$3.P$4 14.86,31.29 v14.86,34.67 | C51.2 3.4,30.76 v2.86,31.3 1.65,32.51 1.65,34.8 2.54,35.69 X3.2 | R27.1 27.49,67.69 25.4,67.69 24.85,67.14 R28.1 23.94,67.69 21.78,67.69 21.23,67.14 R26.2 20.38,67.69 18.61,67.69 18.06,67.14 R25.2 16.87,67.14 16.26,67.75 14.92,67.75 14.48,67.31 12.83,67.31 v11.43,65.91 11.43,63.5 v11.68,63.25 | U$5.P$4 14.86,58.98 v14.86,62.36 | C85.2 3.4,58.45 v2.92,58.93 1.65,60.2 1.65,62.48 2.54,63.37 X7.2
  Top 0.813: R21.1 27.49,53.85 25.4,53.85 24.85,53.3 R22.1 23.94,53.85 21.78,53.85 21.23,53.3 R20.2 20.38,53.85 18.61,53.85 18.06,53.3 R19.2 16.87,53.3 16.26,53.91 14.92,53.91 14.48,53.47 12.83,53.47 v11.43,52.07 11.43,49.66 v11.68,49.4 | U$4.P$4 14.86,45.14 v14.86,48.51 | C68.2 3.4,44.6 v2.92,45.09 1.65,46.35 1.65,48.64 2.54,49.53 X4.2 | R33.1 27.49,81.53 25.4,81.53 24.85,80.98 R34.1 23.94,81.53 21.78,81.53 21.23,80.98 R32.2 20.38,81.53 18.61,81.53 18.06,80.98 R31.2 16.87,80.98 16.26,81.6 14.92,81.6 14.48,81.15 12.83,81.15 v11.43,79.76 11.43,77.34 v11.68,77.09 | U$6.P$4 14.86,72.82 v14.86,76.2 | C102.2 3.4,72.29 v2.79,72.9 1.65,74.04 1.65,76.33 2.54,77.22 X8.2 | R39.1 27.49,95.38 25.4,95.38 24.85,94.83 R40.1 23.94,95.38 21.78,95.38 21.23,94.83 R38.2 20.38,95.38 18.61,95.38 18.06,94.83 R37.2 16.87,94.83 16.26,95.44 14.92,95.44 14.48,95 12.83,95 v11.43,93.6 11.43,91.19 v11.68,90.93 | U$7.P$4 14.86,86.67 v14.86,90.04 | C119.2 3.4,86.13 v2.79,86.74 1.65,87.88 1.65,90.17 2.54,91.06 X9.2 | R45.1 60.14,4.83 62.23,4.83 62.78,5.38 R46.1 63.69,4.83 65.85,4.83 66.4,5.38 R44.2 67.25,4.83 69.03,4.83 69.57,5.38 R43.2 70.76,5.38 71.37,4.76 72.71,4.76 73.15,5.21 74.8,5.21 v76.2,6.6 76.2,9.02 v75.95,9.27 | U$8.P$4 72.77,13.54 v72.77,10.16 | U$9.P$3 77.22,42.04 | C184.2 44.71,83.56 45.72,82.55 U$11.3 | 48.64,44.4 48.64,42.42 49.15,41.91 IC3.6 54.48,41.91 56.13,40.26 C188.+ | v48.94,44.7 49.2,44.45 50.42,44.45 54.1,44.45 54.61,44.96 v54.61,48.01 | v2.88,17.48 2.88,17.46 3.18,17.15 | JP10.2 42.8,25.53 41.78,24.51 41.78,17.78 42.55,17.02 43.81,17.02 X14.2
  Top 1.016: X5.1 83.67,23.34 83.34,23.68 JMP3.3 JMP2.3 | 47.24,82.55 U$11.3 | C155.2 87.65,29.32
  Top 1.27: v67.18,48.77 v67.18,44.58 | v69.47,54.48 v69.47,59.69 69.49,59.72 | v67.44,33.78 67.44,34.42
  Bottom 0.254: U1.12 73.74,19.36 74.3,18.8 v74.42,18.8 | v66.04,17.65 66.55,17.65 v68.07,16
  Bottom 0.305: U3.12 43.79,58.95 42.67,60.07 42.67,64.01 43.56,64.9 46.1,64.9
  Bottom 0.406: 46.1,64.9 51.82,64.9 52.32,65.41
  Bottom 0.61: v82.04,56.39 82.04,57.4 81.28,58.17 80.78,58.17 C152.2 80.77,58.16 80.77,62.48 | JMP6.3 v48.94,44.7 JMP5.3 JMP4.3 | v53.59,64.26 53.47,64.26 52.32,65.41 51.44,66.29 51.44,67.31 C182.2 51.18,67.31 49.53,68.96 49.53,69.47 C183.2 49.28,69.59 49.28,69.85 48.01,71.12 v45.09,71.12 | R58.2 49.28,76.83 49.66,76.45 v50.55,76.45 | X15.6 43.94,91.06 44.7,90.3 44.7,83.57 45.72,82.55 U$11.3 | C187.+ 81.79,87.88 79.38,90.3 U$9.P$22 72.4,90.3 C157.2
  Bottom 0.813: C7.2 C12.2 12.71,9.65 v11.43,9.65 9.78,9.65 9.27,10.16 9.27,10.81 L1.2 9.37,10.95 7.62,12.7 7.62,15.11 6.73,16.89 3.47,16.89 v2.88,17.48 | v14.86,6.1 12.57,6.1 v11.68,6.99 11.43,7.24 6.99,7.24 6.86,7.11 X1.2 | IC1.1 88.47,30.43 v87.48,29.44 | C22.2 C27.2 12.71,24.38 v11.43,24.38 9.78,24.38 9.27,24.89 9.27,25.54 L2.2 9.37,25.68 7.62,27.43 7.62,29.84 6.73,30.73 3.43,30.73 v2.86,31.3 | v14.86,20.83 12.57,20.83 v11.68,21.72 11.43,21.97 6.99,21.97 6.86,21.84 X2.2 | C41.2 C46.2 12.71,38.23 v11.43,38.23 9.78,38.23 9.27,38.73 9.27,39.38 L3.2 9.37,39.52 7.62,41.27 7.62,43.94 6.99,44.58 3.43,44.58 v2.92,45.09 | v14.86,34.67 12.57,34.67 v11.68,35.56 11.43,35.81 6.99,35.81 6.86,35.69 X3.2 | C75.2 C80.2 12.71,65.91 v11.43,65.91 9.78,65.91 9.27,66.42 9.27,67.07 L5.2 9.37,67.21 7.62,68.96 7.62,71.37 6.73,72.26 3.43,72.26 v2.79,72.9 | v14.86,62.36 12.57,62.36 v11.68,63.25 11.43,63.5 6.99,63.5 6.86,63.37 X7.2 | C58.2 C63.2 12.71,52.07 v11.43,52.07 9.78,52.07 9.27,52.58 9.27,53.23 L4.2 9.37,53.37 7.62,55.12 7.62,57.53 6.73,58.42 3.43,58.42 v2.92,58.93 | v14.86,48.51 12.57,48.51 v11.68,49.4 11.43,49.66 6.99,49.66 6.86,49.53 X4.2 | C92.2 C97.2 12.71,79.76 v11.43,79.76 9.78,79.76 9.27,80.26 9.27,80.91 L6.2 9.37,81.05 7.62,82.8 7.62,85.22 6.73,86.11 3.43,86.11 v2.79,86.74 | v14.86,76.2 12.57,76.2 v11.68,77.09 11.43,77.34 6.99,77.34 6.86,77.22 X8.2 | 9.37,94.89 L7.2 9.27,94.76 9.27,94.11 9.78,93.6 v11.43,93.6 12.71,93.6 C114.2 C109.2 | v14.86,90.04 12.57,90.04 v11.68,90.93 11.43,91.19 6.99,91.19 6.86,91.06 X9.2 | 78.26,5.31 L8.2 78.36,5.45 78.36,6.1 77.85,6.6 v76.2,6.6 74.92,6.6 C131.2 C126.2
  Bottom 0.813: v72.77,10.16 75.06,10.16 v75.95,9.27 76.2,9.02 80.64,9.02 80.77,9.14 X10.2 | U$9.P$38 57.66,62.36 56.77,61.47 56.77,54.23 55.12,52.58 55.12,48.51 v54.61,48.01 | X6.2 42.82,8.48 41.66,9.65 41.66,12.83 v41.91,13.08 | v39.62,15.88 41.4,15.88 42.55,17.02 43.81,17.02 X14.2
  Bottom 1.016: 85.45,24.87 85.32,24.74 C40.2 C39.2 85.07,24.74 85.19,24.87 85.45,24.87 | 85.45,24.87 85.95,24.87 X5.1 | R62.1 82.95,62.46 C154.2 80.77,62.48 C153.2 80.65,60.22 R59.2 | C186.2 C185.2 | C185.2 R58.2 | C185.2 U$11.4 U$11.3 | 80.9,31.37 88.92,31.37 IC1.1
  Bottom 1.27: C139.2 44.57,30.48 45.34,29.72 46.61,29.72 | IC4.1 49.4,33.78 49.38,33.76 49.38,29.95 49.15,29.72 | C191.2 U$9.P$3 | v67.18,44.58 v67.18,40.89 C190.1 | v67.18,48.77 69.49,51.08 R66.2 69.47,51.97 v69.47,54.48 | R68.2 69.49,59.72 v69.47,59.69 | 49.15,29.72 46.61,29.72 | JP10.2 45.47,25.53 46.74,26.8 46.74,29.59 46.61,29.72 | 49.15,29.72 50.42,28.45 53.34,28.45 56.13,31.24 C189.- C188.+ 56.13,34.8 57.4,33.53 67.18,33.53 v67.44,33.78
  other vias: 79.12,89.92 68.96,89.03
  pour Top (isolate 0.406): 0.64,98.93 93.6,99.19 93.85,98.68 93.85,1.27 93.98,1.14 0.76,1.14 0.64,1.27
  pour Bottom (isolate 0.406): 0.76,99.19 93.73,99.19 94.11,98.93 93.98,1.52 94.11,1.4 0.89,1.4 0.76,1.52
LFED  (via drill 0.5)
  Top 0.813: C141.2 v80.39,47.5 | v80.14,56.26 77.47,56.26 76.45,57.28 U$9.P$9
  Bottom 0.813: v80.39,47.5 80.39,56.01 v80.14,56.26
LMIX  (via drill 0.5)
  Top 0.406: IC2.2 81.53,45.06 R50.1
  Top 0.813: v38.73,9.02 38.96,8.79 R5.2 40.18,5.94 X6.3 | v38.48,23.75 38.96,23.27 R11.2 39.83,21.89 40.64,20.95 40.64,16.89 43.18,14.35 X14.3 44.91,13.38 46.48,13.38 | v38.48,37.59 38.48,36.22 R17.2 | v38.48,92.96 38.48,91.59 R41.2 | R35.2 38.96,78.64 v38.48,79.12 | R29.2 38.96,64.8 v38.48,65.28 | R23.2 38.96,51.08 v38.48,51.56 | R47.2 46.48,13.38 | 81.53,45.06 83.59,45.06 83.95,44.7 83.95,40.77 84.07,40.64 84.07,33.78 83.31,32.89 77.72,32.89 75.69,30.86 71.75,30.86 67.69,26.8 51.94,26.8 51.56,26.42 50.29,26.42 46.99,23.11 46.99,13.89 46.48,13.38
  Bottom 0.813: v38.73,9.02 38.73,13.34 39.75,14.35 X14.3 | v38.48,23.75 v38.48,37.59 v38.48,51.56 v38.48,65.28 v38.48,79.12 v38.48,92.96
LO1  (via drill 0.5)
  Top 0.61: v79.38,84.2 79.38,85.6 77.22,87.76 77.22,94.87 76.71,95.38 U$9.P$24
  Top 0.813: IC3.1 52.96,35.56 55.12,33.4 61.72,33.4 63.5,35.18 63.5,64.52 63.25,64.77 63.25,79.63 64.14,80.52 64.14,88.01 v64.9,88.77
  Top 1.27: v70.23,97.16 73.28,97.16 U$9.P$24
  Bottom 0.61: IC5.5 80.01,81.53 79.38,82.17 v79.38,84.2
  Bottom 0.813: C146.1 66.55,96.02 66.29,95.76 65.15,94.61 64.9,94.36 v64.9,88.77
  Bottom 1.27: C146.1 v70.23,97.16
LOUT  (via drill 0.5)
  Top 1.27: v61.97,97.16 57.91,97.16 56.64,95.89 X15.1
  Bottom 1.27: C146.2 v61.97,97.16
LP-
  Top 1.016: R71.2 54.38,87.78 U$11.16
  Bottom 0.61: U$11.16 52.07,87.63 C177.2
  Bottom 1.016: C176.1 54.61,87.89 U$11.16
LT
  Bottom 1.016: U$9.P$8 74.55,54.74 72.77,56.52 72.77,61.59 72.01,62.36 72.01,63.5 72.77,64.26 72.77,65.79 71.75,66.8 C175.1
N$1
  Bottom 0.813: X1.3 6.03,9.65 7.62,8.38 11.81,8.38 12.32,7.87 21.46,7.87 C1.1
N$2
  Bottom 0.813: C1.2 24.36,7.77 25.53,6.6 25.53,5.33 26.29,4.57 26.8,4.57 27.3,4.06 27.3,2.72 U$1.P$11 U$1.P$12 U$1.P$13 U$1.P$14
N$3
  Bottom 0.813: X1.1 6.41,4.57 8,6.1 10.79,6.1 12.06,4.83 21.43,4.83 C3.1
N$4
  Bottom 0.813: C3.2 23.84,2.81 U$1.P$9 | U$1.P$7 U$1.P$8 U$1.P$9 | U$1.P$9 U$1.P$10
N$5
  Bottom 0.813: C5.1 33.49,4.87 34.42,3.94 U$1.P$15
N$6
  Bottom 0.813: U$1.P$16 34.39,12.29 32.51,10.41 32.51,6.72 C5.2
N$7
  Bottom 0.813: U$1.P$17 32.61,12.42 31.37,11.18 31.37,8.38 30.23,7.24 30.23,5.21 29.97,4.95 29.07,4.95 C6.1
N$8
  Bottom 0.813: U$1.P$18 30.84,12.29 30.23,11.68 30.23,8.76 29.59,8.13 29.08,8.13 28.96,8 28.96,6.64 C6.2
N$9
  Bottom 0.813: U$1.P$27 14.83,11.47 C7.1
N$10
  Bottom 0.813: U$1.P$26 16.61,11.19 C8.1
N$11
  Bottom 0.813: U$1.P$25 18.39,11.19 C9.1
N$12
  Bottom 0.813: U$1.P$23 21.95,11.19 C10.1
N$13
  Bottom 0.813: U$1.P$24 20.17,11.19 C11.1
N$14
  Bottom 0.813: U$1.P$28 13.06,11.21 C12.1
N$15
  Bottom 0.813: U$1.P$19 29.06,11.19 C13.1
N$16
  Bottom 0.813: U$1.P$20 27.28,11.19 C14.1
N$17
  Bottom 0.813: U$1.P$21 25.5,11.19 C15.1
N$18
  Bottom 0.813: U$1.P$22 23.72,11.19 C16.1
N$19  (via drill 0.5)
  Top 0.813: C17.1 6.58,2.82 v7.21,3.45 | v10.26,4.85 11.3,3.81 U$1.P$2
  Bottom 0.813: v7.21,3.45 8.13,4.45 8.53,4.85 v10.26,4.85
N$20  (via drill 0.5)
  Top 0.813: R1.1 16.86,8.98 v15.62,10.29
  Bottom 0.813: C9.2 C8.2 16.13,9.4 15.75,9.78 v15.62,10.29
N$21  (via drill 0.5)
  Top 0.813: R2.1 20.48,8.98 v19.18,10.29
  Bottom 0.813: C10.2 C11.2 20.21,9.4 19.68,9.4 19.18,9.91 v19.18,10.29
N$22  (via drill 0.5)
  Top 0.813: v26.29,10.22 27.3,9.14 27.88,9.14 R3.2
  Bottom 0.813: C14.2 C13.2 27.06,9.39 v26.29,10.22
N$23  (via drill 0.5)
  Top 0.813: R4.2 24.04,8.98 v22.73,10.29
  Bottom 0.813: C15.2 C16.2 23.24,9.4 22.73,9.91 v22.73,10.29
N$24
  Top 0.406: U$1.P$30 5.69,13.36 JP2.1
N$25
  Top 0.406: U$1.P$1 9.5,3.65 8.32,4.83 7.62,4.83 6.99,5.46 6.99,10.16 6.03,11.11 4.13,11.11 2.98,12.26 2.98,13.14 JP2.2
N$26
  Bottom 0.813: U$1.P$29 11.28,11.52 L1.1
N$27
  Top 0.813: C18.1 35.84,7.14 33.53,4.83 19.18,4.83 18.54,4.19 18.54,2.85 U$1.P$6
N$28
  Top 0.813: C19.1 35.84,9.42 32.38,5.97 17.65,5.97 16.64,4.95 16.64,2.72 U$1.P$5
N$29
  Top 0.813: C18.2 38.94,4.34 R5.1
N$30
  Top 0.813: R6.1 36.7,12.24 C19.2
N$31
  Bottom 0.813: C2.2 24.36,22.5 25.53,21.34 25.53,20.07 26.29,19.3 26.8,19.3 27.3,18.8 27.3,17.45 U$2.P$11 U$2.P$12 U$2.P$13 U$2.P$14
N$32
  Bottom 0.813: C4.2 23.84,17.54 U$2.P$9 | U$2.P$7 U$2.P$8 U$2.P$9 | U$2.P$9 U$2.P$10
N$33
  Bottom 0.813: C20.1 33.49,19.6 34.42,18.67 U$2.P$15
N$34
  Bottom 0.813: U$2.P$16 34.39,26.64 33.66,25.91 33.66,22.39 C20.2
N$35
  Bottom 0.813: U$2.P$17 32.61,26.52 32.38,26.29 32.38,22.99 32,22.61 31.75,22.61 31.37,22.23 31.37,19.94 30.99,19.56 29.02,19.56 C21.1
N$36
  Bottom 0.813: C21.2 29.73,21.35 30.23,21.84 30.23,22.61 30.99,23.37 30.99,27.94 U$2.P$18
N$37
  Bottom 0.813: U$2.P$27 14.83,26.2 C22.1
N$38
  Bottom 0.813: U$2.P$26 16.61,25.92 C23.1
N$39
  Bottom 0.813: U$2.P$25 18.39,25.92 C24.1
N$40
  Bottom 0.813: U$2.P$23 21.95,25.92 C25.1
N$41
  Bottom 0.813: U$2.P$24 20.17,25.92 C26.1
N$42
  Bottom 0.813: U$2.P$28 13.06,25.95 C27.1
N$43
  Bottom 0.813: U$2.P$19 29.06,25.92 C28.1
N$44
  Bottom 0.813: U$2.P$20 27.28,25.92 C29.1
N$45
  Bottom 0.813: U$2.P$21 25.5,25.92 C30.1
N$46
  Bottom 0.813: U$2.P$22 23.72,25.92 C31.1
N$47  (via drill 0.5)
  Top 0.813: C32.1 6.58,17.55 v7.21,18.19 | v10.26,19.58 11.3,18.54 U$2.P$2
  Bottom 0.813: v7.21,18.19 8.13,19.18 8.53,19.58 v10.26,19.58
N$48  (via drill 0.5)
  Top 0.813: R7.1 16.86,23.71 v15.62,25.02
  Bottom 0.813: C24.2 C23.2 16.13,24.13 15.75,24.51 v15.62,25.02
N$49  (via drill 0.5)
  Top 0.813: R8.1 20.48,23.71 v19.18,25.02
  Bottom 0.813: C25.2 C26.2 20.21,24.13 19.68,24.13 19.18,24.64 v19.18,25.02
N$50  (via drill 0.5)
  Top 0.813: v26.29,24.96 27.3,23.88 27.88,23.88 R9.2
  Bottom 0.813: C29.2 C28.2 27.06,24.12 v26.29,24.96
N$51  (via drill 0.5)
  Top 0.813: R10.2 24.04,23.71 v22.73,25.02
  Bottom 0.813: C30.2 C31.2 23.24,24.13 22.73,24.64 v22.73,25.02
N$52
  Top 0.813: C33.1 35.84,21.87 33.53,19.56 19.18,19.56 18.54,18.92 18.54,17.58 U$2.P$6
N$53
  Top 0.813: C34.1 35.84,24.15 32.38,20.7 17.65,20.7 16.64,19.68 16.64,17.45 U$2.P$5
N$54
  Top 0.813: C33.2 38.94,19.07 R11.1
N$55
  Top 0.813: R12.1 36.7,26.97 C34.2
N$56
  Bottom 0.813: X2.1 6.41,19.3 8,20.83 10.79,20.83 12.06,19.56 21.43,19.56 C4.1
N$57
  Top 0.406: U$2.P$30 5.69,28.09 JP3.1
N$58
  Top 0.406: U$2.P$1 9.5,18.38 8.32,19.56 7.62,19.56 6.99,20.19 6.99,24.89 6.03,25.84 4.13,25.84 2.98,26.99 2.98,27.88 JP3.2
N$59
  Bottom 0.813: X2.3 6.03,24.38 7.62,23.11 11.81,23.11 12.32,22.61 21.46,22.61 C2.1
N$60
  Bottom 0.813: U$2.P$29 11.28,26.25 L2.1
N$61
  Bottom 0.813: C35.2 24.36,36.35 25.53,35.18 25.53,33.91 26.29,33.15 26.8,33.15 27.3,32.64 27.3,31.29 U$3.P$11 U$3.P$12 U$3.P$13 U$3.P$14
N$62
  Bottom 0.813: C36.2 23.84,31.38 U$3.P$9 | U$3.P$7 U$3.P$8 U$3.P$9 | U$3.P$9 U$3.P$10
N$63
  Bottom 0.813: C37.1 33.49,33.44 34.42,32.51 U$3.P$15
N$64
  Bottom 0.813: U$3.P$16 34.39,40.49 33.66,39.75 33.66,36.23 C37.2
N$65
  Bottom 0.813: U$3.P$17 32.61,40.36 32.38,40.13 32.38,36.83 32,36.45 31.75,36.45 31.37,36.07 31.37,33.78 30.99,33.4 29.02,33.4 C38.1
N$66
  Bottom 0.813: C38.2 29.73,35.19 30.23,35.69 30.23,36.45 30.99,37.21 30.99,41.78 U$3.P$18
N$67
  Bottom 0.813: U$3.P$27 14.83,40.04 C41.1
N$68
  Bottom 0.813: U$3.P$26 16.61,39.76 C42.1
N$69
  Bottom 0.813: U$3.P$25 18.39,39.76 C43.1
N$70
  Bottom 0.813: U$3.P$23 21.95,39.76 C44.1
N$71
  Bottom 0.813: U$3.P$24 20.17,39.76 C45.1
N$72
  Bottom 0.813: U$3.P$28 13.06,39.79 C46.1
N$73
  Bottom 0.813: U$3.P$19 29.06,39.76 C47.1
N$74
  Bottom 0.813: U$3.P$20 27.28,39.76 C48.1
N$75
  Bottom 0.813: U$3.P$21 25.5,39.76 C49.1
N$76
  Bottom 0.813: U$3.P$22 23.72,39.76 C50.1
N$77  (via drill 0.5)
  Top 0.813: C51.1 6.58,31.4 v7.21,32.03 | v10.26,33.43 11.3,32.38 U$3.P$2
  Bottom 0.813: v7.21,32.03 8.13,33.02 8.53,33.43 v10.26,33.43
N$78  (via drill 0.5)
  Top 0.813: R13.1 16.86,37.56 v15.62,38.86
  Bottom 0.813: C43.2 C42.2 16.65,37.97 16.13,37.97 15.75,38.35 v15.62,38.86
N$79  (via drill 0.5)
  Top 0.813: R14.1 20.48,37.56 v19.18,38.86
  Bottom 0.813: C44.2 C45.2 20.21,37.97 19.68,37.97 19.18,38.48 v19.18,38.86
N$80  (via drill 0.5)
  Top 0.813: v26.29,38.8 27.3,37.72 27.88,37.72 R15.2
  Bottom 0.813: C48.2 C47.2 27.06,37.96 v26.29,38.8
N$81  (via drill 0.5)
  Top 0.813: R16.2 24.04,37.56 v22.73,38.86
  Bottom 0.813: C49.2 C50.2 23.76,37.97 23.24,37.97 22.73,38.48 v22.73,38.86
N$82
  Top 0.813: C52.1 35.84,35.72 33.53,33.4 19.18,33.4 18.54,32.77 18.54,31.42 U$3.P$6
N$83
  Top 0.813: C53.1 35.84,37.99 32.38,34.54 17.65,34.54 16.64,33.53 16.64,31.29 U$3.P$5
N$84
  Top 0.813: C52.2 38.94,32.91 R17.1
N$85
  Top 0.813: R18.1 36.7,40.82 C53.2
N$86
  Bottom 0.813: X3.1 6.41,33.15 8,34.67 10.79,34.67 12.06,33.4 21.43,33.4 C36.1
N$87
  Top 0.406: U$3.P$30 5.69,41.94 JP4.1
N$88
  Top 0.406: U$3.P$1 9.5,32.22 8.32,33.4 7.62,33.4 6.99,34.04 6.99,38.73 6.03,39.69 4.13,39.69 2.98,40.83 2.98,41.72 JP4.2
N$89
  Bottom 0.813: X3.3 6.03,38.23 7.62,36.96 11.81,36.96 12.32,36.45 21.46,36.45 C35.1
N$90
  Bottom 0.813: U$3.P$29 11.28,40.09 L3.1
N$91
  Bottom 0.813: C54.2 24.36,50.19 25.53,49.02 25.53,47.75 26.29,46.99 26.8,46.99 27.3,46.48 27.3,45.14 U$4.P$11 U$4.P$12 U$4.P$13 U$4.P$14
N$92
  Bottom 0.813: C55.2 23.84,45.22 U$4.P$9 | U$4.P$7 U$4.P$8 U$4.P$9 | U$4.P$9 U$4.P$10
N$93
  Bottom 0.813: C56.1 33.49,47.28 34.42,46.35 U$4.P$15
N$94
  Bottom 0.813: U$4.P$16 34.39,54.33 33.66,53.59 33.66,50.08 C56.2
N$95
  Bottom 0.813: U$4.P$17 32.61,54.2 32.38,53.98 32.38,50.67 32,50.29 31.75,50.29 31.37,49.91 31.37,47.62 30.99,47.24 29.02,47.24 C57.1
N$96
  Bottom 0.813: C57.2 29.73,49.03 30.23,49.53 30.23,50.29 30.99,51.05 30.99,55.63 U$4.P$18
N$97
  Bottom 0.813: U$4.P$27 14.83,53.88 C58.1
N$98
  Bottom 0.813: U$4.P$26 16.61,53.6 C59.1
N$99
  Bottom 0.813: U$4.P$25 18.39,53.6 C60.1
N$100
  Bottom 0.813: U$4.P$23 21.95,53.6 C61.1
N$101
  Bottom 0.813: U$4.P$24 20.17,53.6 C62.1
N$102
  Bottom 0.813: U$4.P$28 13.06,53.63 C63.1
N$103
  Bottom 0.813: U$4.P$19 29.06,53.6 C64.1
N$104
  Bottom 0.813: U$4.P$20 27.28,53.6 C65.1
N$105
  Bottom 0.813: U$4.P$21 25.5,53.6 C66.1
N$106
  Bottom 0.813: U$4.P$22 23.72,53.6 C67.1
N$107  (via drill 0.5)
  Top 0.813: C68.1 6.58,45.24 v7.21,45.87 | v10.26,47.27 11.3,46.23 U$4.P$2
  Bottom 0.813: v7.21,45.87 8.13,46.86 8.53,47.27 v10.26,47.27
N$108  (via drill 0.5)
  Top 0.813: R19.1 16.86,51.4 v15.62,52.7
  Bottom 0.813: C60.2 C59.2 16.65,51.82 16.13,51.82 15.75,52.2 v15.62,52.7
N$109  (via drill 0.5)
  Top 0.813: R20.1 20.48,51.4 v19.18,52.7
  Bottom 0.813: C61.2 C62.2 20.21,51.82 19.68,51.82 19.18,52.32 v19.18,52.7
N$110  (via drill 0.5)
  Top 0.813: v26.29,52.64 27.3,51.56 27.88,51.56 R21.2
  Bottom 0.813: C65.2 C64.2 27.06,51.8 v26.29,52.64
N$111  (via drill 0.5)
  Top 0.813: R22.2 24.04,51.4 v22.73,52.7
  Bottom 0.813: C66.2 C67.2 23.76,51.82 23.24,51.82 22.73,52.32 v22.73,52.7
N$112
  Top 0.813: C69.1 35.84,49.56 33.53,47.24 19.18,47.24 18.54,46.61 18.54,45.26 U$4.P$6
N$113
  Top 0.813: C70.1 35.84,51.84 32.38,48.39 17.65,48.39 16.64,47.37 16.64,45.14 U$4.P$5
N$114
  Top 0.813: C69.2 38.94,46.76 R23.1
N$115
  Top 0.813: R24.1 36.7,54.66 C70.2
N$116
  Bottom 0.813: X4.1 6.41,46.99 8,48.51 10.79,48.51 12.06,47.24 21.43,47.24 C55.1
N$117
  Top 0.406: U$4.P$30 5.69,55.78 JP5.1
N$118
  Top 0.406: U$4.P$1 9.5,46.06 8.32,47.24 7.62,47.24 6.99,47.88 6.99,52.58 6.03,53.53 4.13,53.53 2.98,54.67 2.98,55.56 JP5.2
N$119
  Bottom 0.813: X4.3 6.03,52.07 7.62,50.8 11.81,50.8 12.32,50.29 21.46,50.29 C54.1
N$120
  Bottom 0.813: U$4.P$29 11.28,53.94 L4.1
N$121
  Bottom 0.813: C71.2 24.36,64.03 25.53,62.87 25.53,61.59 26.29,60.83 26.8,60.83 27.3,60.33 27.3,58.98 U$5.P$11 U$5.P$12 U$5.P$13 U$5.P$14
N$122
  Bottom 0.813: C72.2 23.84,59.07 U$5.P$9 | U$5.P$7 U$5.P$8 U$5.P$9 | U$5.P$9 U$5.P$10
N$123
  Bottom 0.813: C73.1 33.49,61.13 34.42,60.2 U$5.P$15
N$124
  Bottom 0.813: U$5.P$16 34.39,68.17 33.66,67.44 33.66,63.92 C73.2
N$125
  Bottom 0.813: U$5.P$17 32.61,68.05 32.38,67.82 32.38,64.52 32,64.14 31.75,64.14 31.37,63.75 31.37,61.47 30.99,61.09 29.02,61.09 C74.1
N$126
  Bottom 0.813: C74.2 29.73,62.88 30.23,63.37 30.23,64.39 30.99,65.15 30.99,69.47 U$5.P$18
N$127
  Bottom 0.813: U$5.P$27 14.83,67.73 C75.1
N$128
  Bottom 0.813: U$5.P$26 16.61,67.45 C76.1
N$129
  Bottom 0.813: U$5.P$25 18.39,67.45 C77.1
N$130
  Bottom 0.813: U$5.P$23 21.95,67.45 C78.1
N$131
  Bottom 0.813: U$5.P$24 20.17,67.45 C79.1
N$132
  Bottom 0.813: U$5.P$28 13.06,67.47 C80.1
N$133
  Bottom 0.813: U$5.P$19 29.06,67.45 C81.1
N$134
  Bottom 0.813: U$5.P$20 27.28,67.45 C82.1
N$135
  Bottom 0.813: U$5.P$21 25.5,67.45 C83.1
N$136
  Bottom 0.813: U$5.P$22 23.72,67.45 C84.1
N$137  (via drill 0.5)
  Top 0.813: C85.1 6.58,59.08 v7.21,59.72 | v10.26,61.11 11.3,60.07 U$5.P$2
  Bottom 0.813: v7.21,59.72 8.13,60.71 8.53,61.11 v10.26,61.11
N$138  (via drill 0.5)
  Top 0.813: R25.1 16.86,65.24 v15.62,66.55
  Bottom 0.813: C77.2 C76.2 16.13,65.66 15.75,66.04 v15.62,66.55
N$139  (via drill 0.5)
  Top 0.813: R26.1 20.48,65.24 v19.18,66.55
  Bottom 0.813: C78.2 C79.2 20.21,65.66 19.68,65.66 19.18,66.17 v19.18,66.55
N$140  (via drill 0.5)
  Top 0.813: v26.29,66.48 27.3,65.41 27.88,65.41 R27.2
  Bottom 0.813: C82.2 C81.2 27.06,65.65 v26.29,66.48
N$141  (via drill 0.5)
  Top 0.813: R28.2 24.04,65.24 v22.73,66.55
  Bottom 0.813: C83.2 C84.2 23.24,65.66 22.73,66.17 v22.73,66.55
N$142
  Top 0.813: C86.1 35.84,63.4 33.53,61.09 19.18,61.09 18.54,60.45 18.54,59.11 U$5.P$6
N$143
  Top 0.813: C87.1 35.84,65.68 32.38,62.23 17.65,62.23 16.64,61.21 16.64,58.98 U$5.P$5
N$144
  Top 0.813: C86.2 38.94,60.6 R29.1
N$145
  Top 0.813: R30.1 36.7,68.5 C87.2
N$146
  Bottom 0.813: X7.1 6.41,60.83 8,62.36 10.79,62.36 12.06,61.09 21.43,61.09 C72.1
N$147
  Top 0.406: U$5.P$30 5.69,69.62 JP6.1
N$148
  Top 0.406: U$5.P$1 9.5,59.91 8.32,61.09 7.62,61.09 6.99,61.72 6.99,66.42 6.03,67.37 4.13,67.37 2.98,68.52 2.98,69.41 JP6.2
N$149
  Bottom 0.813: X7.3 6.03,65.91 7.62,64.64 11.81,64.64 12.32,64.14 21.46,64.14 C71.1
N$150
  Bottom 0.813: U$5.P$29 11.28,67.78 L5.1
N$151
  Bottom 0.813: C88.2 24.36,77.88 25.53,76.71 25.53,75.44 26.29,74.68 26.8,74.68 27.3,74.17 27.3,72.82 U$6.P$11 U$6.P$12 U$6.P$13 U$6.P$14
N$152
  Bottom 0.813: C89.2 23.84,72.91 U$6.P$9 | U$6.P$7 U$6.P$8 U$6.P$9 | U$6.P$9 U$6.P$10
N$153
  Bottom 0.813: C90.1 33.49,74.97 34.42,74.04 U$6.P$15
N$154
  Bottom 0.813: U$6.P$16 34.39,82.02 33.66,81.28 33.66,77.76 C90.2
N$155
  Bottom 0.813: U$6.P$17 32.61,81.89 32.38,81.66 32.38,78.36 32,77.98 31.75,77.98 31.37,77.6 31.37,75.31 30.99,74.93 29.02,74.93 C91.1
N$156
  Bottom 0.813: C91.2 29.73,76.72 30.23,77.22 30.23,77.98 30.99,78.74 30.99,83.31 U$6.P$18
N$157
  Bottom 0.813: U$6.P$27 14.83,81.57 C92.1
N$158
  Bottom 0.813: U$6.P$26 16.61,81.29 C93.1
N$159
  Bottom 0.813: U$6.P$25 18.39,81.29 C94.1
N$160
  Bottom 0.813: U$6.P$23 21.95,81.29 C95.1
N$161
  Bottom 0.813: U$6.P$24 20.17,81.29 C96.1
N$162
  Bottom 0.813: U$6.P$28 13.06,81.32 C97.1
N$163
  Bottom 0.813: U$6.P$19 29.06,81.29 C98.1
N$164
  Bottom 0.813: U$6.P$20 27.28,81.29 C99.1
N$165
  Bottom 0.813: U$6.P$21 25.5,81.29 C100.1
N$166
  Bottom 0.813: U$6.P$22 23.72,81.29 C101.1
N$167  (via drill 0.5)
  Top 0.813: C102.1 6.58,72.93 v7.21,73.56 | v10.26,74.95 11.3,73.91 U$6.P$2
  Bottom 0.813: v7.21,73.56 8.13,74.55 8.53,74.95 v10.26,74.95
N$168  (via drill 0.5)
  Top 0.813: R31.1 16.86,79.08 v15.62,80.39
  Bottom 0.813: C94.2 C93.2 16.65,79.5 16.13,79.5 15.75,79.88 v15.62,80.39
N$169  (via drill 0.5)
  Top 0.813: R32.1 20.48,79.08 v19.18,80.39
  Bottom 0.813: C95.2 C96.2 20.21,79.5 19.68,79.5 19.18,80.01 v19.18,80.39
N$170  (via drill 0.5)
  Top 0.813: v26.29,80.33 27.3,79.25 27.88,79.25 R33.2
  Bottom 0.813: C99.2 C98.2 27.06,79.49 v26.29,80.33
N$171  (via drill 0.5)
  Top 0.813: R34.2 24.04,79.08 v22.73,80.39
  Bottom 0.813: C100.2 C101.2 23.76,79.5 23.24,79.5 22.73,80.01 v22.73,80.39
N$172
  Top 0.813: C103.1 35.84,77.24 33.53,74.93 19.18,74.93 18.54,74.3 18.54,72.95 U$6.P$6
N$173
  Top 0.813: C104.1 35.84,79.52 32.38,76.07 17.65,76.07 16.64,75.06 16.64,72.82 U$6.P$5
N$174
  Top 0.813: C103.2 38.94,74.44 R35.1
N$175
  Top 0.813: R36.1 36.7,82.35 C104.2
N$176
  Bottom 0.813: X8.1 6.41,74.68 8,76.2 10.79,76.2 12.06,74.93 21.43,74.93 C89.1
N$177
  Top 0.406: U$6.P$30 5.69,83.46 JP7.1
N$178
  Top 0.406: U$6.P$1 9.5,73.75 8.32,74.93 7.62,74.93 6.99,75.56 6.99,80.26 6.03,81.22 4.13,81.22 2.98,82.36 2.98,83.25 JP7.2
N$179
  Bottom 0.813: X8.3 6.03,79.76 7.62,78.49 11.81,78.49 12.32,77.98 21.46,77.98 C88.1
N$180
  Bottom 0.813: U$6.P$29 11.28,81.62 L6.1
N$181
  Bottom 0.813: C105.2 24.36,91.72 25.53,90.55 25.53,89.28 26.29,88.52 26.8,88.52 27.3,88.01 27.3,86.67 U$7.P$11 U$7.P$12 U$7.P$13 U$7.P$14
N$182
  Bottom 0.813: C106.2 23.84,86.75 U$7.P$9 | U$7.P$7 U$7.P$8 U$7.P$9 | U$7.P$9 U$7.P$10
N$183
  Bottom 0.813: C107.1 33.49,88.81 34.42,87.88 U$7.P$15
N$184
  Bottom 0.813: U$7.P$16 34.39,95.86 33.66,95.12 33.66,91.6 C107.2
N$185
  Bottom 0.813: U$7.P$17 32.61,95.73 32.38,95.5 32.38,92.2 32,91.82 31.75,91.82 31.37,91.44 31.37,89.15 30.99,88.77 29.02,88.77 C108.1
N$186
  Bottom 0.813: C108.2 29.73,90.56 30.23,91.06 30.23,91.82 30.99,92.58 30.99,97.16 U$7.P$18
N$187
  Bottom 0.813: U$7.P$27 14.83,95.41 C109.1
N$188
  Bottom 0.813: U$7.P$26 16.61,95.13 C110.1
N$189
  Bottom 0.813: U$7.P$25 18.39,95.13 C111.1
N$190
  Bottom 0.813: U$7.P$23 21.95,95.13 C112.1
N$191
  Bottom 0.813: U$7.P$24 20.17,95.13 C113.1
N$192
  Bottom 0.813: U$7.P$28 13.06,95.16 C114.1
N$193
  Bottom 0.813: U$7.P$19 29.06,95.13 C115.1
N$194
  Bottom 0.813: U$7.P$20 27.28,95.13 C116.1
N$195
  Bottom 0.813: U$7.P$21 25.5,95.13 C117.1
N$196
  Bottom 0.813: U$7.P$22 23.72,95.13 C118.1
N$197  (via drill 0.5)
  Top 0.813: C119.1 6.58,86.77 v7.21,87.4 | v10.26,88.8 11.3,87.76 U$7.P$2
  Bottom 0.813: v7.21,87.4 8.13,88.39 8.53,88.8 v10.26,88.8
N$198  (via drill 0.5)
  Top 0.813: R37.1 16.86,92.93 v15.62,94.23
  Bottom 0.813: C111.2 C110.2 16.65,93.34 16.13,93.34 15.75,93.73 v15.62,94.23
N$199  (via drill 0.5)
  Top 0.813: R38.1 20.48,92.93 v19.18,94.23
  Bottom 0.813: C112.2 C113.2 20.21,93.34 19.68,93.34 19.18,93.85 v19.18,94.23
N$200  (via drill 0.5)
  Top 0.813: v26.29,94.17 27.3,93.09 27.88,93.09 R39.2
  Bottom 0.813: C116.2 C115.2 27.06,93.33 v26.29,94.17
N$201  (via drill 0.5)
  Top 0.813: R40.2 24.04,92.93 v22.73,94.23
